(* Logix 5000 Program export KEP; software revision 30.00; part 12 of 15 *)
(* tags used below, declared in another part *)
   B256_CtoE : B256_CtoE;
   B256_CtoS : B256_CtoS;
   B256_EtoC : B256_EtoC;
   B256_StoC_LE : B256_StoC_LE;
   B256_StoSLE : B256_StoSLE;
   EdDSA_INTERNAL : EdDSA_INTERNAL[5];
   EdDSA_STATES : EdDSA_STATECTRL[15];
   InternalFlags : InternalFlags[5];
   InternalFlag_KeyServerIdentityNo : BOOL;
   InternalFlag_KeyServerIdentityYes : BOOL;
   InternalFlag_KsExists : BOOL;
   InternalFlag_KsIDMatchesServer : BOOL;
   InternalFlag_KsPrimeExists : BOOL;
   InternalFlag_KsPrimeIDMatchesServer : BOOL;
   InternalFlag_PowerOnCycle : BOOL;
   MyNodeNumber : DINT;
   POINT_ENC : POINT_ENC;
   POINT_MUL : POINT_MUL;
   PRN : STRING;
   PRNG : PRNG;
   PRNG_Constant : STRING;
   PRNG_Counter : LINT;
   PRNG_Seed : LINT[13];
   ServerNode : INT;
   ServerPriority : DINT[5];
   SignedMsgDest : INT;   // 0=None 1=Server 2=Client 3=All
   Temp_Processor_C1 : DINT[22];
   Temp_Processor_C10 : DINT[22];
   Temp_Processor_C2 : DINT[22];
   Temp_Processor_C3 : DINT[22];
   Temp_Processor_C4 : DINT[22];
   Temp_Processor_C5 : DINT[22];
   Temp_Processor_C6 : DINT[22];
   Temp_Processor_C7 : DINT[22];
   Temp_Processor_C8 : DINT[22];
   Temp_Processor_C9 : DINT[22];
   Temp_Processor_D1 : DINT[43];
   Temp_Processor_E1 : DINT[32];
   Temp_Processor_E2 : DINT[32];
   Temp_Processor_HASH : LINT[8];
   Temp_Processor_L : LINT[4];
   Temp_Processor_MSG : LINT[1600];
   Temp_Processor_P1 : POINT;
   Temp_Processor_P2 : POINT;
   Temp_Processor_P3 : POINT;
   Temp_Processor_P4 : POINT;
   Temp_Processor_S : STRING;
   T_INT1 : INT;
   WorkingNode : DINT;
   NODE : VMAC_DATA_INTERNAL[5];
(* KEP, continued *)

ROUTINE PROCESSOR_STATE1   (* ladder *)
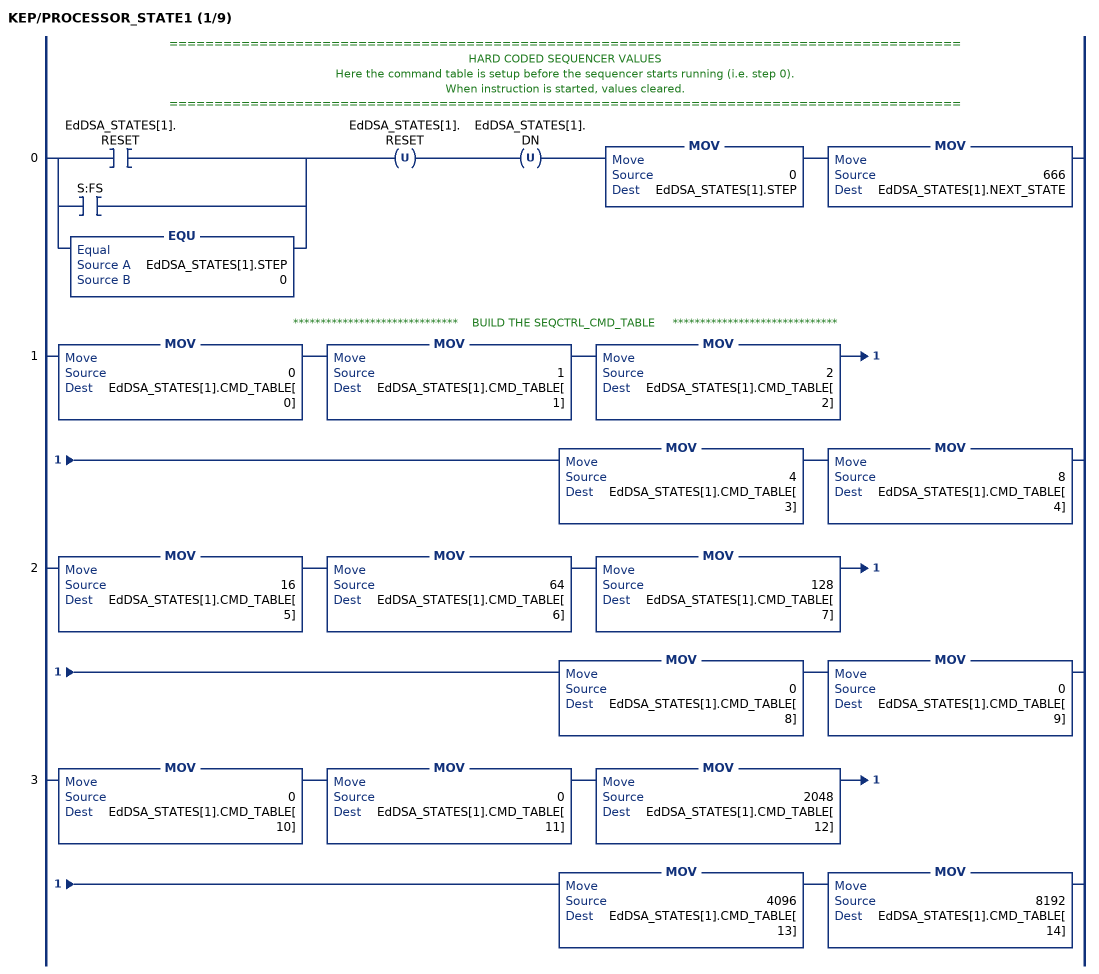
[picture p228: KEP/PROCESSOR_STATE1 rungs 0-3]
   // ========================================================================================
   // HARD CODED SEQUENCER VALUES
   // Here the command table is setup before the sequencer starts running (i.e. step 0).
   // When instruction is started, values cleared.
   // ========================================================================================
   0: [[XIC(EdDSA_STATES[1].RESET) ,XIC(S:FS) ] ,EQU(EdDSA_STATES[1].STEP,0) ]OTU(EdDSA_STATES[1].RESET)OTU(EdDSA_STATES[1].DN)MOV(0,EdDSA_STATES[1].STEP)MOV(666,EdDSA_STATES[1].NEXT_STATE);
   // ******************************    BUILD THE SEQCTRL_CMD_TABLE     ******************************
   1: MOV(0,EdDSA_STATES[1].CMD_TABLE[0])MOV(1,EdDSA_STATES[1].CMD_TABLE[1])MOV(2,EdDSA_STATES[1].CMD_TABLE[2])MOV(4,EdDSA_STATES[1].CMD_TABLE[3])MOV(8,EdDSA_STATES[1].CMD_TABLE[4]);
   2: MOV(16,EdDSA_STATES[1].CMD_TABLE[5])MOV(64,EdDSA_STATES[1].CMD_TABLE[6])MOV(128,EdDSA_STATES[1].CMD_TABLE[7])MOV(0,EdDSA_STATES[1].CMD_TABLE[8])MOV(0,EdDSA_STATES[1].CMD_TABLE[9]);
   3: MOV(0,EdDSA_STATES[1].CMD_TABLE[10])MOV(0,EdDSA_STATES[1].CMD_TABLE[11])MOV(2048,EdDSA_STATES[1].CMD_TABLE[12])MOV(4096,EdDSA_STATES[1].CMD_TABLE[13])MOV(8192,EdDSA_STATES[1].CMD_TABLE[14]);
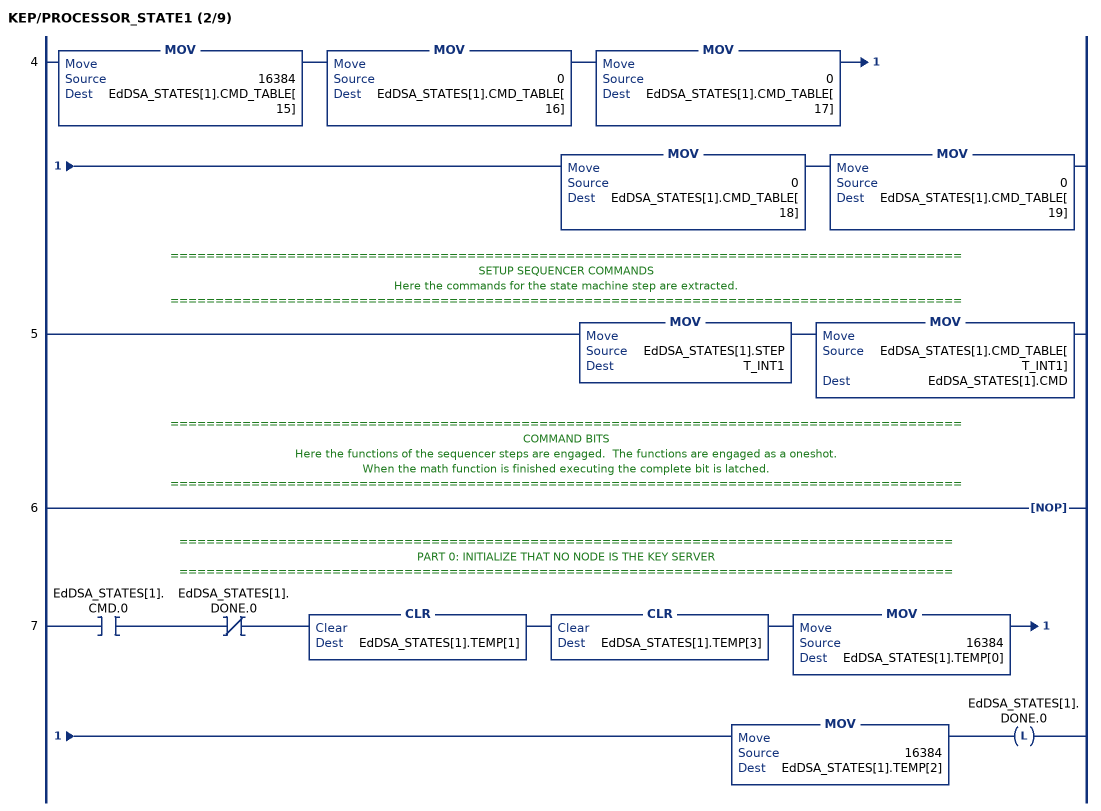
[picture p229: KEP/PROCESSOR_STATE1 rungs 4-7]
   4: MOV(16384,EdDSA_STATES[1].CMD_TABLE[15])MOV(0,EdDSA_STATES[1].CMD_TABLE[16])MOV(0,EdDSA_STATES[1].CMD_TABLE[17])MOV(0,EdDSA_STATES[1].CMD_TABLE[18])MOV(0,EdDSA_STATES[1].CMD_TABLE[19]);
   // ========================================================================================
   // SETUP SEQUENCER COMMANDS
   // Here the commands for the state machine step are extracted.
   // ========================================================================================
   5: MOV(EdDSA_STATES[1].STEP,T_INT1)MOV(EdDSA_STATES[1].CMD_TABLE[T_INT1],EdDSA_STATES[1].CMD);
   // ========================================================================================
   // COMMAND BITS
   // Here the functions of the sequencer steps are engaged.  The functions are engaged as a oneshot.
   // When the math function is finished executing the complete bit is latched.
   // ========================================================================================
   6: NOP();
   // ======================================================================================
   // PART 0: INITIALIZE THAT NO NODE IS THE KEY SERVER
   // ======================================================================================
   7: XIC(EdDSA_STATES[1].CMD.0)XIO(EdDSA_STATES[1].DONE.0)CLR(EdDSA_STATES[1].TEMP[1])CLR(EdDSA_STATES[1].TEMP[3])MOV(16384,EdDSA_STATES[1].TEMP[0])MOV(16384,EdDSA_STATES[1].TEMP[2])OTL(EdDSA_STATES[1].DONE.0);
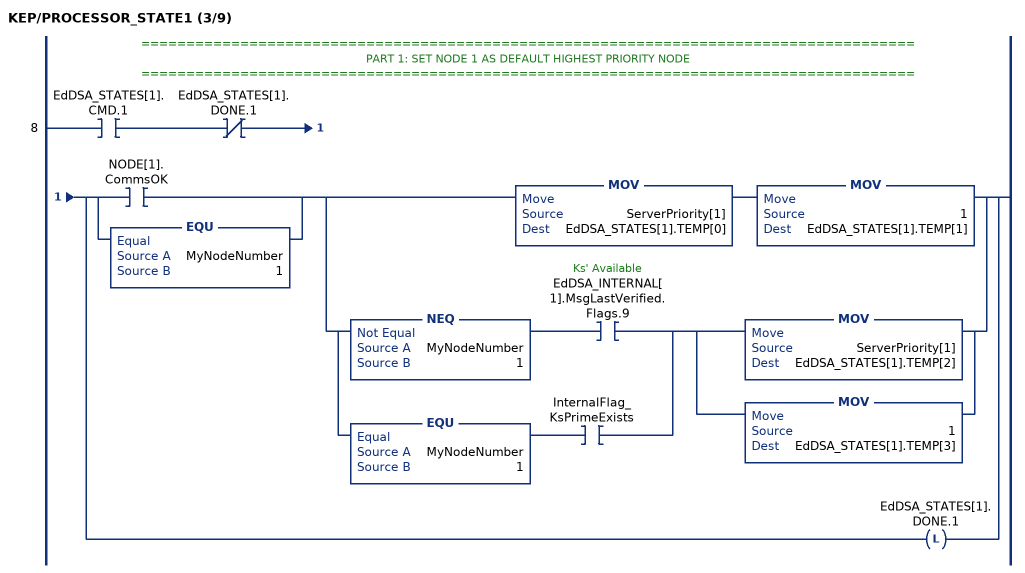
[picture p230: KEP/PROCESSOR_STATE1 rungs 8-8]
   // ======================================================================================
   // PART 1: SET NODE 1 AS DEFAULT HIGHEST PRIORITY NODE
   // ======================================================================================
   8: XIC(EdDSA_STATES[1].CMD.1)XIO(EdDSA_STATES[1].DONE.1)[[XIC(NODE[1].CommsOK) ,EQU(MyNodeNumber,1) ] [MOV(ServerPriority[1],EdDSA_STATES[1].TEMP[0]) MOV(1,EdDSA_STATES[1].TEMP[1]) ,[NEQ(MyNodeNumber,1) XIC(EdDSA_INTERNAL[1].MsgLastVerified.Flags.9) ,EQU(MyNodeNumber,1) XIC(InternalFlag_KsPrimeExists) ] [MOV(ServerPriority[1],EdDSA_STATES[1].TEMP[2]) ,MOV(1,EdDSA_STATES[1].TEMP[3]) ] ] ,OTL(EdDSA_STATES[1].DONE.1) ];
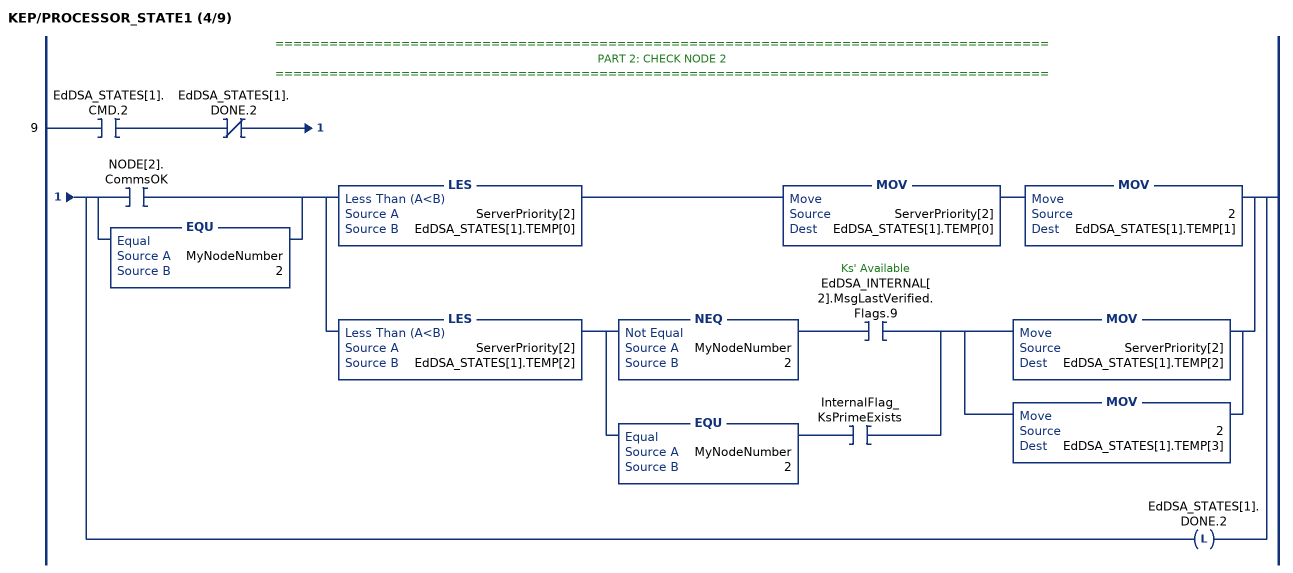
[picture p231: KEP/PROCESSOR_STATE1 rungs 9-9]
   // ======================================================================================
   // PART 2: CHECK NODE 2
   // ======================================================================================
   9: XIC(EdDSA_STATES[1].CMD.2)XIO(EdDSA_STATES[1].DONE.2)[[XIC(NODE[2].CommsOK) ,EQU(MyNodeNumber,2) ] [LES(ServerPriority[2],EdDSA_STATES[1].TEMP[0]) MOV(ServerPriority[2],EdDSA_STATES[1].TEMP[0]) MOV(2,EdDSA_STATES[1].TEMP[1]) ,LES(ServerPriority[2],EdDSA_STATES[1].TEMP[2]) [NEQ(MyNodeNumber,2) XIC(EdDSA_INTERNAL[2].MsgLastVerified.Flags.9) ,EQU(MyNodeNumber,2) XIC(InternalFlag_KsPrimeExists) ] [MOV(ServerPriority[2],EdDSA_STATES[1].TEMP[2]) ,MOV(2,EdDSA_STATES[1].TEMP[3]) ] ] ,OTL(EdDSA_STATES[1].DONE.2) ];
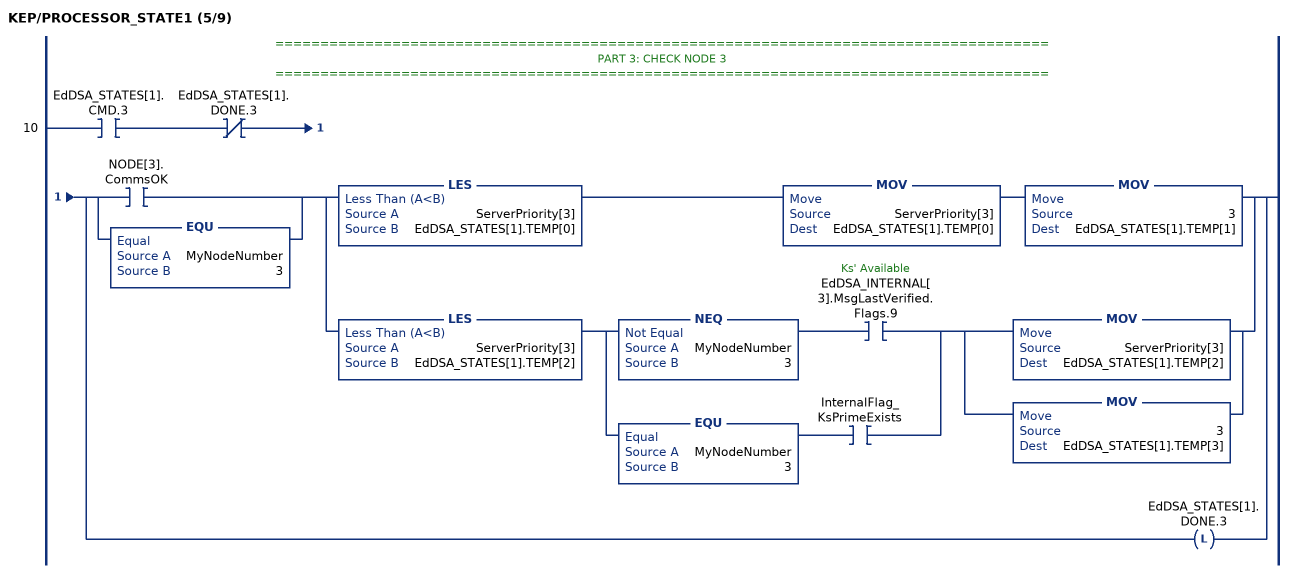
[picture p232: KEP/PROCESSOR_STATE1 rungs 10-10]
   // ======================================================================================
   // PART 3: CHECK NODE 3
   // ======================================================================================
   10: XIC(EdDSA_STATES[1].CMD.3)XIO(EdDSA_STATES[1].DONE.3)[[XIC(NODE[3].CommsOK) ,EQU(MyNodeNumber,3) ] [LES(ServerPriority[3],EdDSA_STATES[1].TEMP[0]) MOV(ServerPriority[3],EdDSA_STATES[1].TEMP[0]) MOV(3,EdDSA_STATES[1].TEMP[1]) ,LES(ServerPriority[3],EdDSA_STATES[1].TEMP[2]) [NEQ(MyNodeNumber,3) XIC(EdDSA_INTERNAL[3].MsgLastVerified.Flags.9) ,EQU(MyNodeNumber,3) XIC(InternalFlag_KsPrimeExists) ] [MOV(ServerPriority[3],EdDSA_STATES[1].TEMP[2]) ,MOV(3,EdDSA_STATES[1].TEMP[3]) ] ] ,OTL(EdDSA_STATES[1].DONE.3) ];
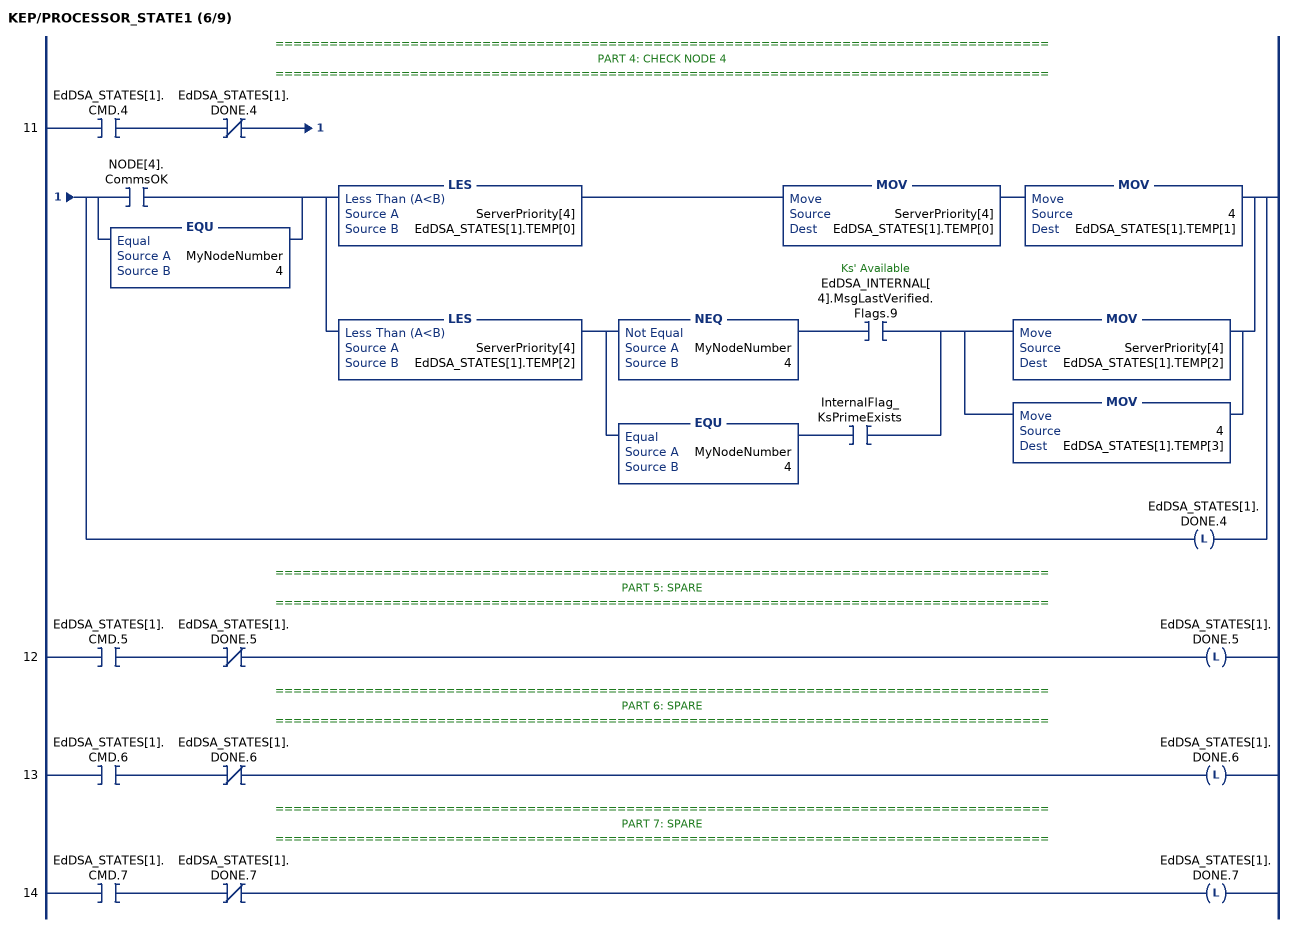
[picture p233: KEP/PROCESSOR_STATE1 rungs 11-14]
   // ======================================================================================
   // PART 4: CHECK NODE 4
   // ======================================================================================
   11: XIC(EdDSA_STATES[1].CMD.4)XIO(EdDSA_STATES[1].DONE.4)[[XIC(NODE[4].CommsOK) ,EQU(MyNodeNumber,4) ] [LES(ServerPriority[4],EdDSA_STATES[1].TEMP[0]) MOV(ServerPriority[4],EdDSA_STATES[1].TEMP[0]) MOV(4,EdDSA_STATES[1].TEMP[1]) ,LES(ServerPriority[4],EdDSA_STATES[1].TEMP[2]) [NEQ(MyNodeNumber,4) XIC(EdDSA_INTERNAL[4].MsgLastVerified.Flags.9) ,EQU(MyNodeNumber,4) XIC(InternalFlag_KsPrimeExists) ] [MOV(ServerPriority[4],EdDSA_STATES[1].TEMP[2]) ,MOV(4,EdDSA_STATES[1].TEMP[3]) ] ] ,OTL(EdDSA_STATES[1].DONE.4) ];
   // ======================================================================================
   // PART 5: SPARE
   // ======================================================================================
   12: XIC(EdDSA_STATES[1].CMD.5)XIO(EdDSA_STATES[1].DONE.5)OTL(EdDSA_STATES[1].DONE.5);
   // ======================================================================================
   // PART 6: SPARE
   // ======================================================================================
   13: XIC(EdDSA_STATES[1].CMD.6)XIO(EdDSA_STATES[1].DONE.6)OTL(EdDSA_STATES[1].DONE.6);
   // ======================================================================================
   // PART 7: SPARE
   // ======================================================================================
   14: XIC(EdDSA_STATES[1].CMD.7)XIO(EdDSA_STATES[1].DONE.7)OTL(EdDSA_STATES[1].DONE.7);
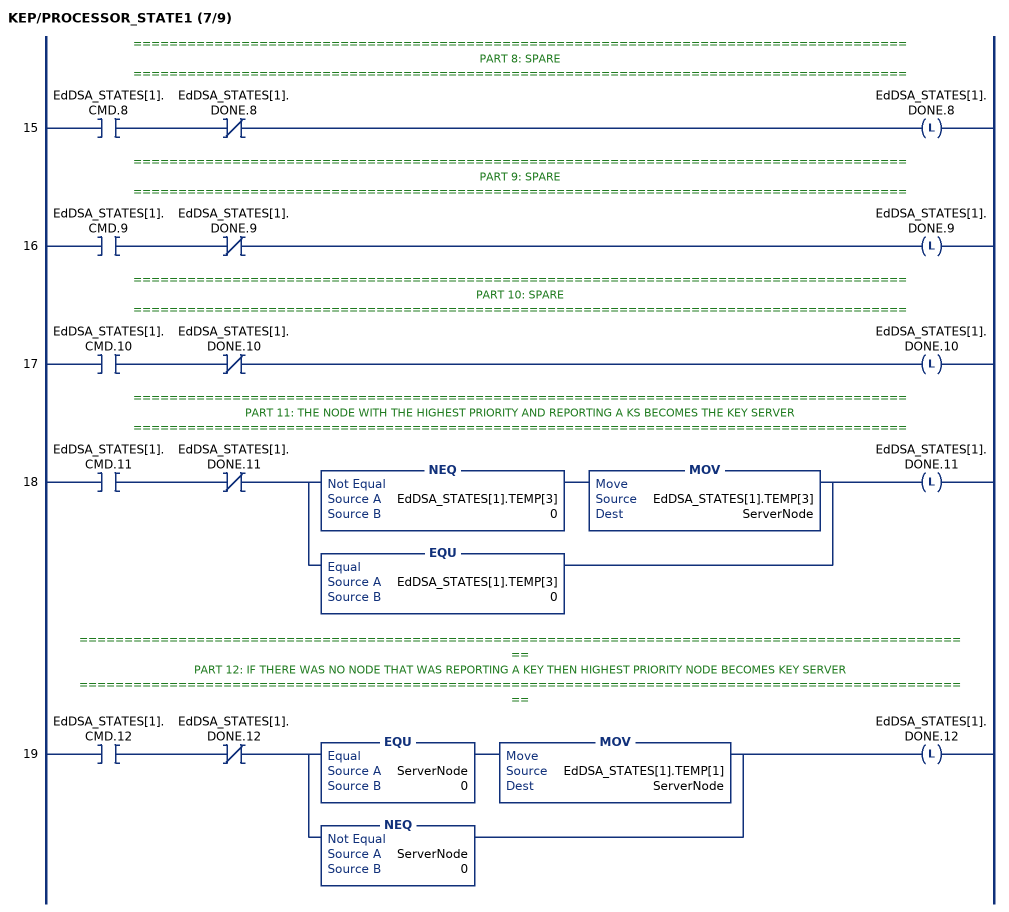
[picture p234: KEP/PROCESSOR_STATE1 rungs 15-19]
   // ======================================================================================
   // PART 8: SPARE
   // ======================================================================================
   15: XIC(EdDSA_STATES[1].CMD.8)XIO(EdDSA_STATES[1].DONE.8)OTL(EdDSA_STATES[1].DONE.8);
   // ======================================================================================
   // PART 9: SPARE
   // ======================================================================================
   16: XIC(EdDSA_STATES[1].CMD.9)XIO(EdDSA_STATES[1].DONE.9)OTL(EdDSA_STATES[1].DONE.9);
   // ======================================================================================
   // PART 10: SPARE
   // ======================================================================================
   17: XIC(EdDSA_STATES[1].CMD.10)XIO(EdDSA_STATES[1].DONE.10)OTL(EdDSA_STATES[1].DONE.10);
   // ======================================================================================
   // PART 11: THE NODE WITH THE HIGHEST PRIORITY AND REPORTING A KS BECOMES THE KEY SERVER
   // ======================================================================================
   18: XIC(EdDSA_STATES[1].CMD.11)XIO(EdDSA_STATES[1].DONE.11)[NEQ(EdDSA_STATES[1].TEMP[3],0) MOV(EdDSA_STATES[1].TEMP[3],ServerNode) ,EQU(EdDSA_STATES[1].TEMP[3],0) ]OTL(EdDSA_STATES[1].DONE.11);
   // ====================================================================================================
   // PART 12: IF THERE WAS NO NODE THAT WAS REPORTING A KEY THEN HIGHEST PRIORITY NODE BECOMES KEY SERVER
   // ====================================================================================================
   19: XIC(EdDSA_STATES[1].CMD.12)XIO(EdDSA_STATES[1].DONE.12)[EQU(ServerNode,0) MOV(EdDSA_STATES[1].TEMP[1],ServerNode) ,NEQ(ServerNode,0) ]OTL(EdDSA_STATES[1].DONE.12);
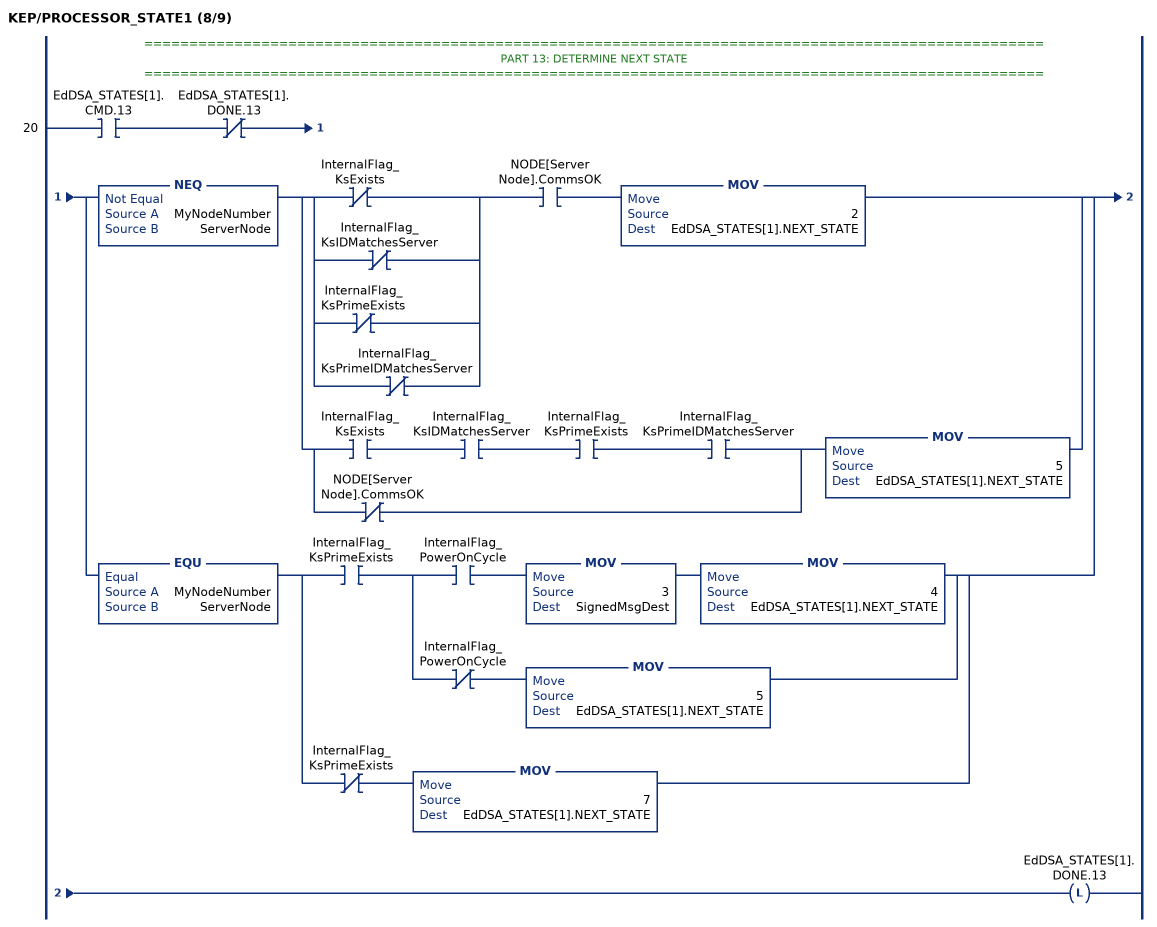
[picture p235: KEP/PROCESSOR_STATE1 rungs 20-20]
   // ====================================================================================================
   // PART 13: DETERMINE NEXT STATE
   // ====================================================================================================
   20: XIC(EdDSA_STATES[1].CMD.13)XIO(EdDSA_STATES[1].DONE.13)[NEQ(MyNodeNumber,ServerNode) [[XIO(InternalFlag_KsExists) ,XIO(InternalFlag_KsIDMatchesServer) ,XIO(InternalFlag_KsPrimeExists) ,XIO(InternalFlag_KsPrimeIDMatchesServer) ] XIC(NODE[ServerNode].CommsOK) MOV(2,EdDSA_STATES[1].NEXT_STATE) ,[XIC(InternalFlag_KsExists) XIC(InternalFlag_KsIDMatchesServer) XIC(InternalFlag_KsPrimeExists) XIC(InternalFlag_KsPrimeIDMatchesServer) ,XIO(NODE[ServerNode].CommsOK) ] MOV(5,EdDSA_STATES[1].NEXT_STATE) ] ,EQU(MyNodeNumber,ServerNode) [XIC(InternalFlag_KsPrimeExists) [XIC(InternalFlag_PowerOnCycle) MOV(3,SignedMsgDest) MOV(4,EdDSA_STATES[1].NEXT_STATE) ,XIO(InternalFlag_PowerOnCycle) MOV(5,EdDSA_STATES[1].NEXT_STATE) ] ,XIO(InternalFlag_KsPrimeExists) MOV(7,EdDSA_STATES[1].NEXT_STATE) ] ]OTL(EdDSA_STATES[1].DONE.13);
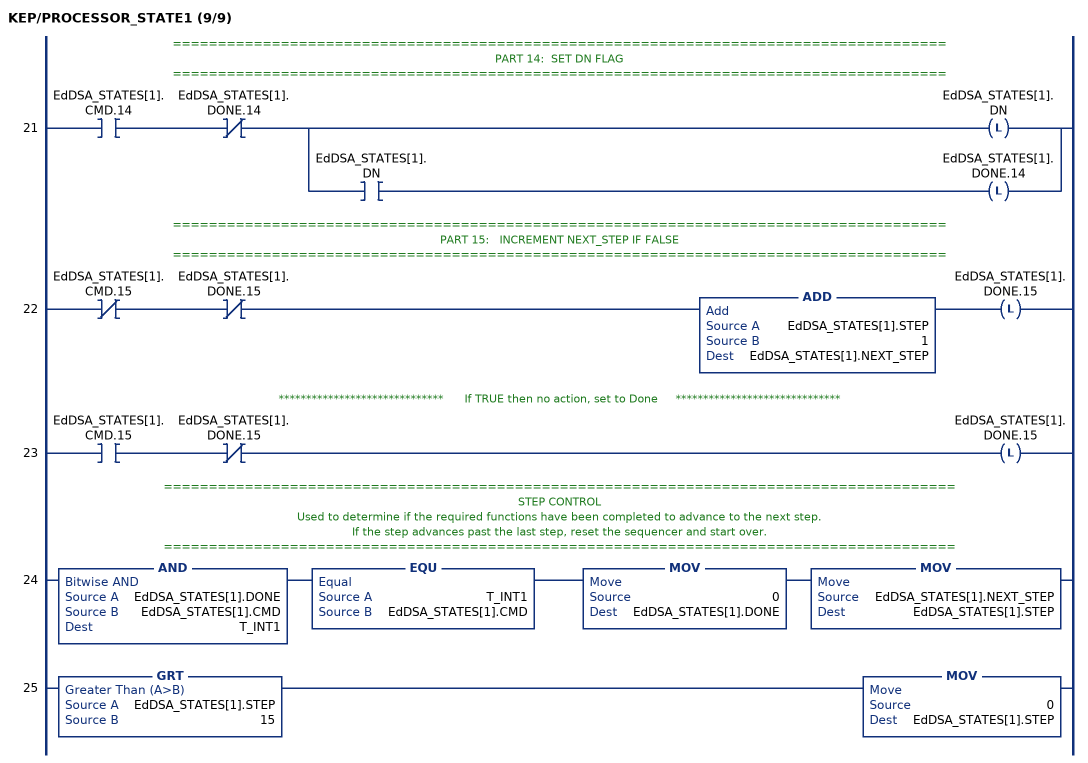
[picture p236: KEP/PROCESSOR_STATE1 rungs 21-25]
   // ======================================================================================
   // PART 14:  SET DN FLAG
   // ======================================================================================
   21: XIC(EdDSA_STATES[1].CMD.14)XIO(EdDSA_STATES[1].DONE.14)[OTL(EdDSA_STATES[1].DN) ,XIC(EdDSA_STATES[1].DN) OTL(EdDSA_STATES[1].DONE.14) ];
   // ======================================================================================
   // PART 15:   INCREMENT NEXT_STEP IF FALSE
   // ======================================================================================
   22: XIO(EdDSA_STATES[1].CMD.15)XIO(EdDSA_STATES[1].DONE.15)ADD(EdDSA_STATES[1].STEP,1,EdDSA_STATES[1].NEXT_STEP)OTL(EdDSA_STATES[1].DONE.15);
   // ******************************      If TRUE then no action, set to Done     ******************************
   23: XIC(EdDSA_STATES[1].CMD.15)XIO(EdDSA_STATES[1].DONE.15)OTL(EdDSA_STATES[1].DONE.15);
   // ========================================================================================
   // STEP CONTROL
   // Used to determine if the required functions have been completed to advance to the next step.
   // If the step advances past the last step, reset the sequencer and start over.
   // ========================================================================================
   24: AND(EdDSA_STATES[1].DONE,EdDSA_STATES[1].CMD,T_INT1)EQU(T_INT1,EdDSA_STATES[1].CMD)MOV(0,EdDSA_STATES[1].DONE)MOV(EdDSA_STATES[1].NEXT_STEP,EdDSA_STATES[1].STEP);
   25: GRT(EdDSA_STATES[1].STEP,15)MOV(0,EdDSA_STATES[1].STEP);
END_ROUTINE

ROUTINE PROCESSOR_STATE2   (* ladder *)
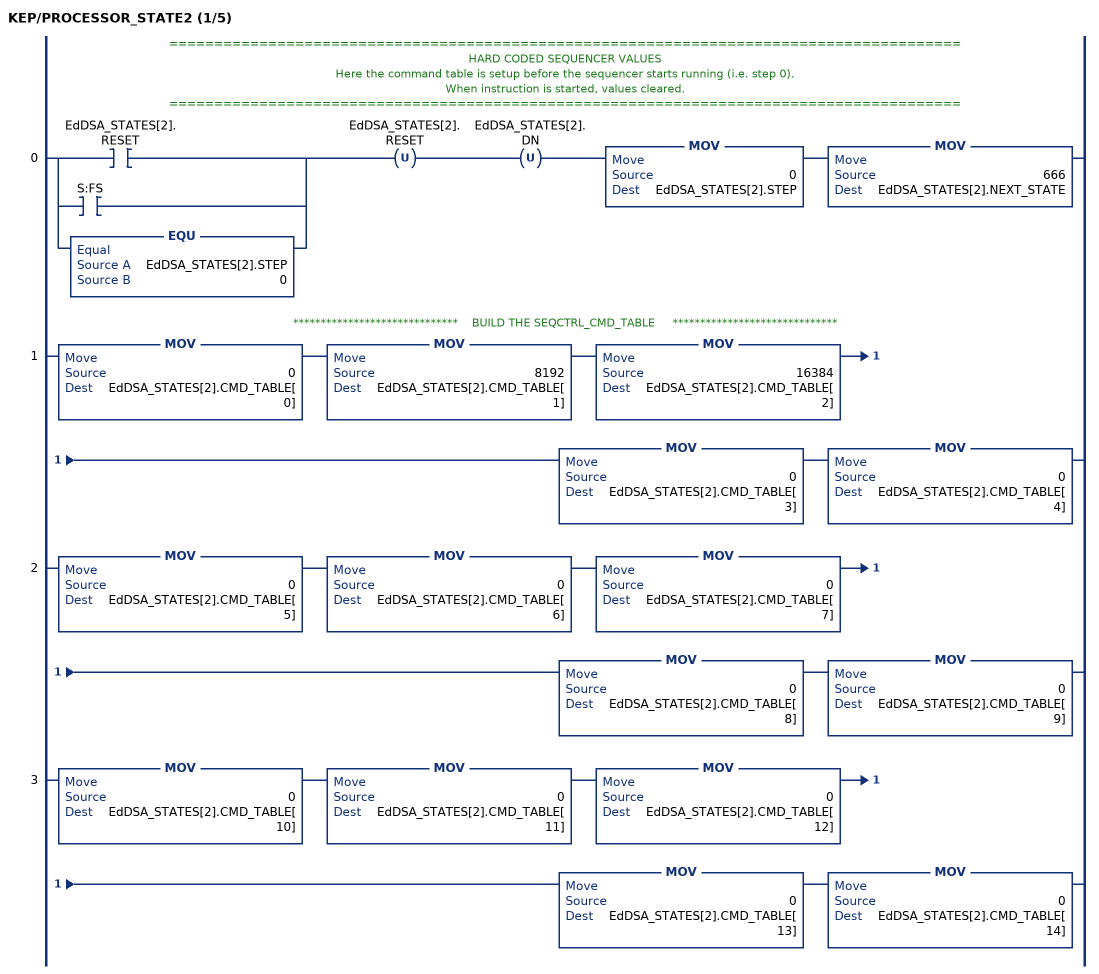
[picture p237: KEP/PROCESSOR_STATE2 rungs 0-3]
   // ========================================================================================
   // HARD CODED SEQUENCER VALUES
   // Here the command table is setup before the sequencer starts running (i.e. step 0).
   // When instruction is started, values cleared.
   // ========================================================================================
   0: [[XIC(EdDSA_STATES[2].RESET) ,XIC(S:FS) ] ,EQU(EdDSA_STATES[2].STEP,0) ]OTU(EdDSA_STATES[2].RESET)OTU(EdDSA_STATES[2].DN)MOV(0,EdDSA_STATES[2].STEP)MOV(666,EdDSA_STATES[2].NEXT_STATE);
   // ******************************    BUILD THE SEQCTRL_CMD_TABLE     ******************************
   1: MOV(0,EdDSA_STATES[2].CMD_TABLE[0])MOV(8192,EdDSA_STATES[2].CMD_TABLE[1])MOV(16384,EdDSA_STATES[2].CMD_TABLE[2])MOV(0,EdDSA_STATES[2].CMD_TABLE[3])MOV(0,EdDSA_STATES[2].CMD_TABLE[4]);
   2: MOV(0,EdDSA_STATES[2].CMD_TABLE[5])MOV(0,EdDSA_STATES[2].CMD_TABLE[6])MOV(0,EdDSA_STATES[2].CMD_TABLE[7])MOV(0,EdDSA_STATES[2].CMD_TABLE[8])MOV(0,EdDSA_STATES[2].CMD_TABLE[9]);
   3: MOV(0,EdDSA_STATES[2].CMD_TABLE[10])MOV(0,EdDSA_STATES[2].CMD_TABLE[11])MOV(0,EdDSA_STATES[2].CMD_TABLE[12])MOV(0,EdDSA_STATES[2].CMD_TABLE[13])MOV(0,EdDSA_STATES[2].CMD_TABLE[14]);
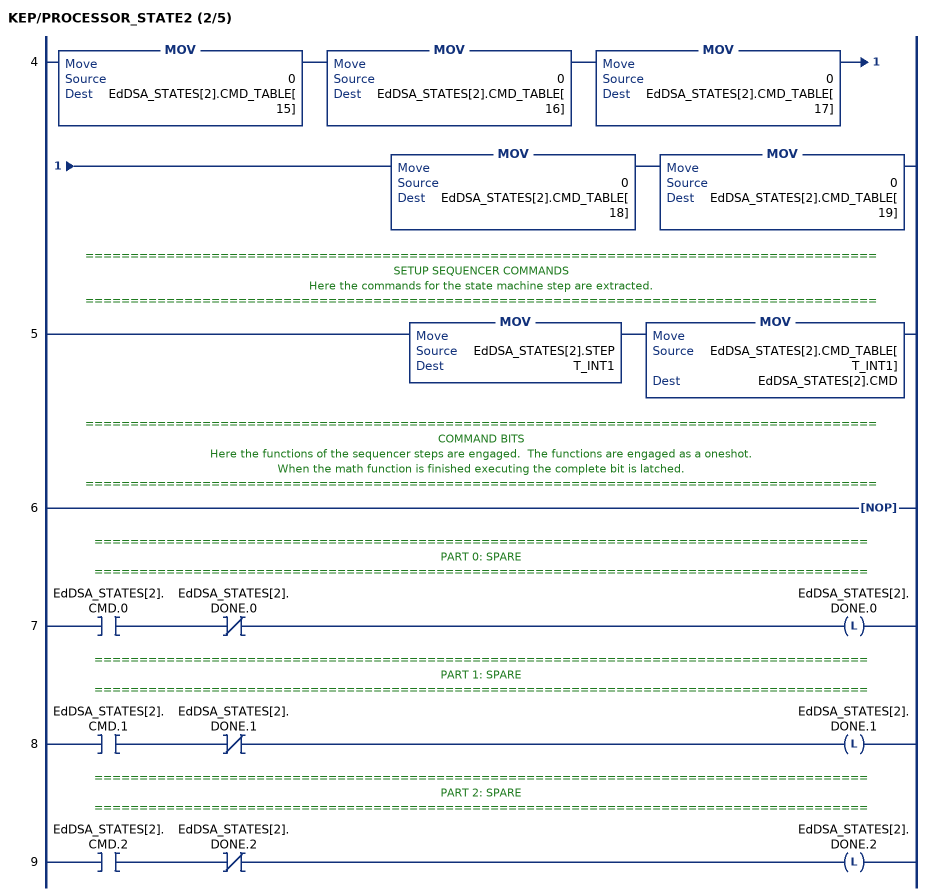
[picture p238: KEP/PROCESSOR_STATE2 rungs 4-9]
   4: MOV(0,EdDSA_STATES[2].CMD_TABLE[15])MOV(0,EdDSA_STATES[2].CMD_TABLE[16])MOV(0,EdDSA_STATES[2].CMD_TABLE[17])MOV(0,EdDSA_STATES[2].CMD_TABLE[18])MOV(0,EdDSA_STATES[2].CMD_TABLE[19]);
   // ========================================================================================
   // SETUP SEQUENCER COMMANDS
   // Here the commands for the state machine step are extracted.
   // ========================================================================================
   5: MOV(EdDSA_STATES[2].STEP,T_INT1)MOV(EdDSA_STATES[2].CMD_TABLE[T_INT1],EdDSA_STATES[2].CMD);
   // ========================================================================================
   // COMMAND BITS
   // Here the functions of the sequencer steps are engaged.  The functions are engaged as a oneshot.
   // When the math function is finished executing the complete bit is latched.
   // ========================================================================================
   6: NOP();
   // ======================================================================================
   // PART 0: SPARE
   // ======================================================================================
   7: XIC(EdDSA_STATES[2].CMD.0)XIO(EdDSA_STATES[2].DONE.0)OTL(EdDSA_STATES[2].DONE.0);
   // ======================================================================================
   // PART 1: SPARE
   // ======================================================================================
   8: XIC(EdDSA_STATES[2].CMD.1)XIO(EdDSA_STATES[2].DONE.1)OTL(EdDSA_STATES[2].DONE.1);
   // ======================================================================================
   // PART 2: SPARE
   // ======================================================================================
   9: XIC(EdDSA_STATES[2].CMD.2)XIO(EdDSA_STATES[2].DONE.2)OTL(EdDSA_STATES[2].DONE.2);
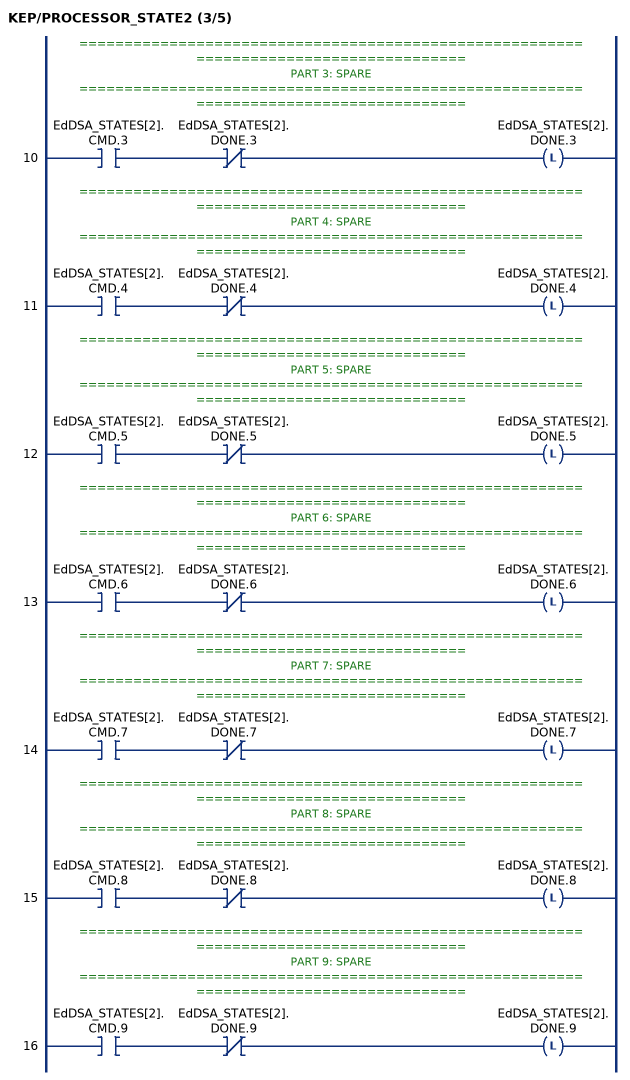
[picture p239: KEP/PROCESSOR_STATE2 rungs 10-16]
   // ======================================================================================
   // PART 3: SPARE
   // ======================================================================================
   10: XIC(EdDSA_STATES[2].CMD.3)XIO(EdDSA_STATES[2].DONE.3)OTL(EdDSA_STATES[2].DONE.3);
   // ======================================================================================
   // PART 4: SPARE
   // ======================================================================================
   11: XIC(EdDSA_STATES[2].CMD.4)XIO(EdDSA_STATES[2].DONE.4)OTL(EdDSA_STATES[2].DONE.4);
   // ======================================================================================
   // PART 5: SPARE
   // ======================================================================================
   12: XIC(EdDSA_STATES[2].CMD.5)XIO(EdDSA_STATES[2].DONE.5)OTL(EdDSA_STATES[2].DONE.5);
   // ======================================================================================
   // PART 6: SPARE
   // ======================================================================================
   13: XIC(EdDSA_STATES[2].CMD.6)XIO(EdDSA_STATES[2].DONE.6)OTL(EdDSA_STATES[2].DONE.6);
   // ======================================================================================
   // PART 7: SPARE
   // ======================================================================================
   14: XIC(EdDSA_STATES[2].CMD.7)XIO(EdDSA_STATES[2].DONE.7)OTL(EdDSA_STATES[2].DONE.7);
   // ======================================================================================
   // PART 8: SPARE
   // ======================================================================================
   15: XIC(EdDSA_STATES[2].CMD.8)XIO(EdDSA_STATES[2].DONE.8)OTL(EdDSA_STATES[2].DONE.8);
   // ======================================================================================
   // PART 9: SPARE
   // ======================================================================================
   16: XIC(EdDSA_STATES[2].CMD.9)XIO(EdDSA_STATES[2].DONE.9)OTL(EdDSA_STATES[2].DONE.9);
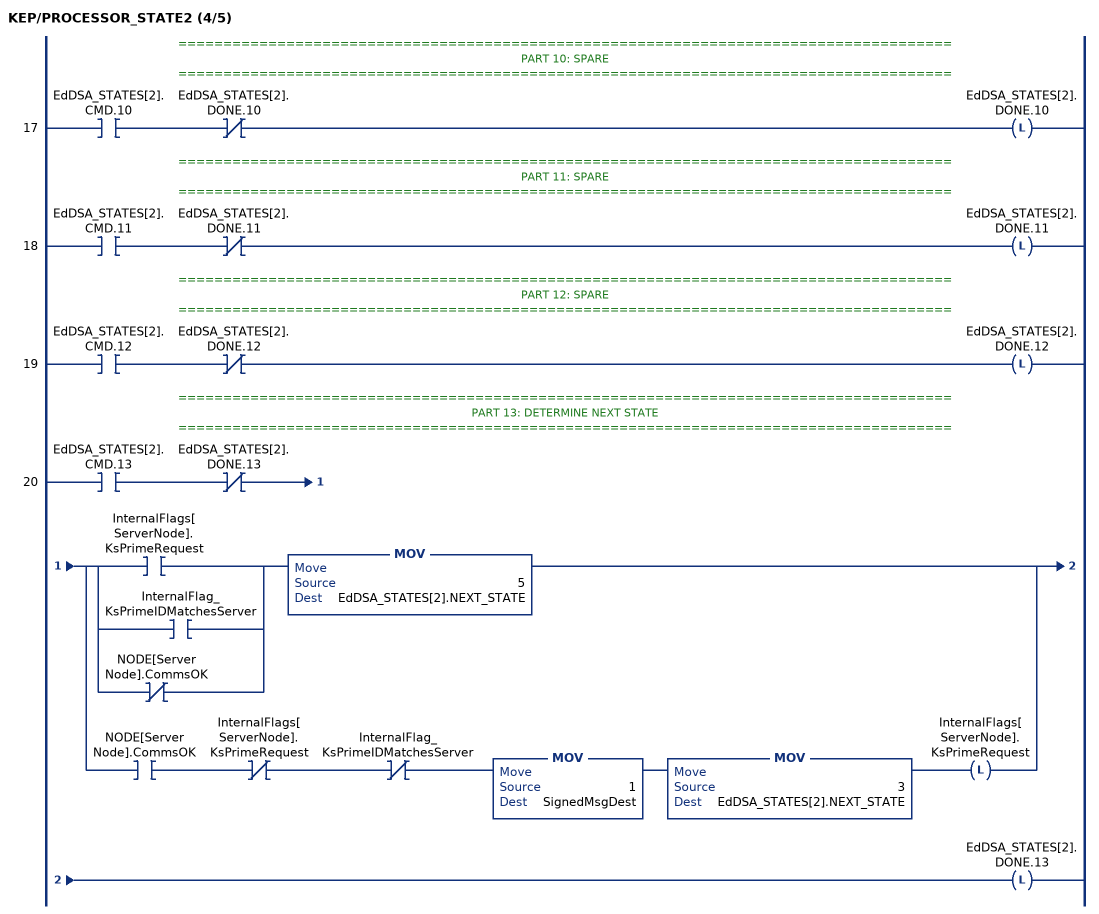
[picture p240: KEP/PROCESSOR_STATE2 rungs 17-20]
   // ======================================================================================
   // PART 10: SPARE
   // ======================================================================================
   17: XIC(EdDSA_STATES[2].CMD.10)XIO(EdDSA_STATES[2].DONE.10)OTL(EdDSA_STATES[2].DONE.10);
   // ======================================================================================
   // PART 11: SPARE
   // ======================================================================================
   18: XIC(EdDSA_STATES[2].CMD.11)XIO(EdDSA_STATES[2].DONE.11)OTL(EdDSA_STATES[2].DONE.11);
   // ======================================================================================
   // PART 12: SPARE
   // ======================================================================================
   19: XIC(EdDSA_STATES[2].CMD.12)XIO(EdDSA_STATES[2].DONE.12)OTL(EdDSA_STATES[2].DONE.12);
   // ======================================================================================
   // PART 13: DETERMINE NEXT STATE
   // ======================================================================================
   20: XIC(EdDSA_STATES[2].CMD.13)XIO(EdDSA_STATES[2].DONE.13)[[XIC(InternalFlags[ServerNode].KsPrimeRequest) ,XIC(InternalFlag_KsPrimeIDMatchesServer) ,XIO(NODE[ServerNode].CommsOK) ] MOV(5,EdDSA_STATES[2].NEXT_STATE) ,XIC(NODE[ServerNode].CommsOK) XIO(InternalFlags[ServerNode].KsPrimeRequest) XIO(InternalFlag_KsPrimeIDMatchesServer) MOV(1,SignedMsgDest) MOV(3,EdDSA_STATES[2].NEXT_STATE) OTL(InternalFlags[ServerNode].KsPrimeRequest) ]OTL(EdDSA_STATES[2].DONE.13);
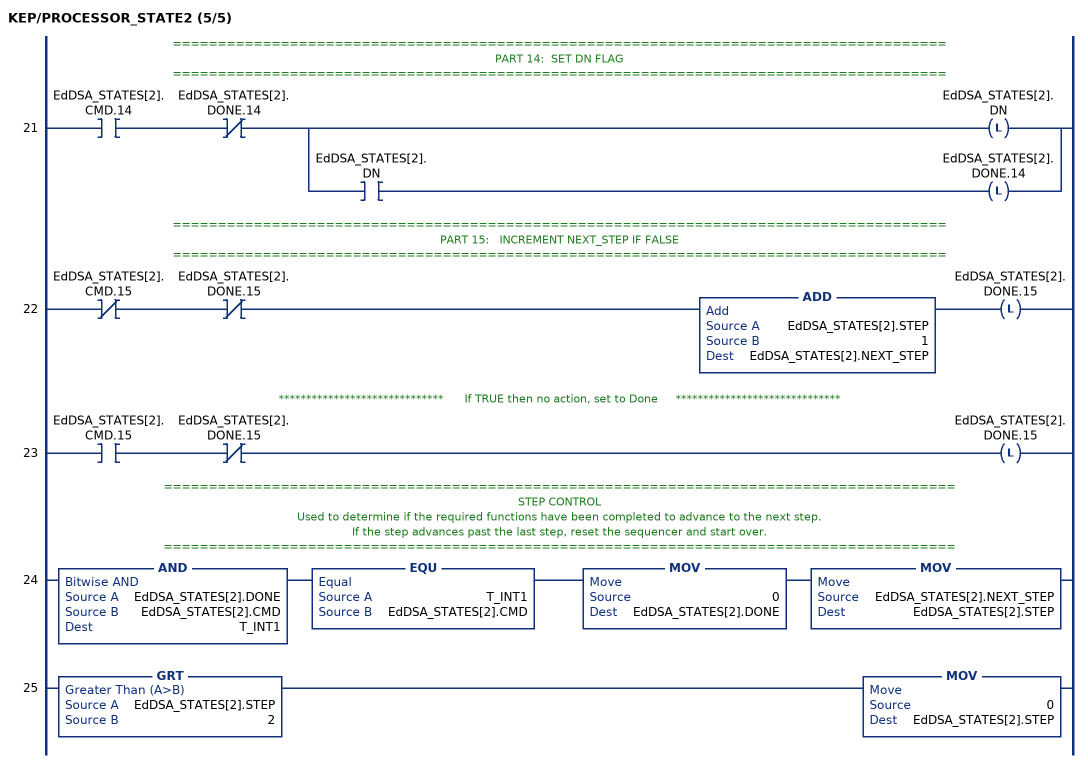
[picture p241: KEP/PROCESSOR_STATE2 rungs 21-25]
   // ======================================================================================
   // PART 14:  SET DN FLAG
   // ======================================================================================
   21: XIC(EdDSA_STATES[2].CMD.14)XIO(EdDSA_STATES[2].DONE.14)[OTL(EdDSA_STATES[2].DN) ,XIC(EdDSA_STATES[2].DN) OTL(EdDSA_STATES[2].DONE.14) ];
   // ======================================================================================
   // PART 15:   INCREMENT NEXT_STEP IF FALSE
   // ======================================================================================
   22: XIO(EdDSA_STATES[2].CMD.15)XIO(EdDSA_STATES[2].DONE.15)ADD(EdDSA_STATES[2].STEP,1,EdDSA_STATES[2].NEXT_STEP)OTL(EdDSA_STATES[2].DONE.15);
   // ******************************      If TRUE then no action, set to Done     ******************************
   23: XIC(EdDSA_STATES[2].CMD.15)XIO(EdDSA_STATES[2].DONE.15)OTL(EdDSA_STATES[2].DONE.15);
   // ========================================================================================
   // STEP CONTROL
   // Used to determine if the required functions have been completed to advance to the next step.
   // If the step advances past the last step, reset the sequencer and start over.
   // ========================================================================================
   24: AND(EdDSA_STATES[2].DONE,EdDSA_STATES[2].CMD,T_INT1)EQU(T_INT1,EdDSA_STATES[2].CMD)MOV(0,EdDSA_STATES[2].DONE)MOV(EdDSA_STATES[2].NEXT_STEP,EdDSA_STATES[2].STEP);
   25: GRT(EdDSA_STATES[2].STEP,2)MOV(0,EdDSA_STATES[2].STEP);
END_ROUTINE

ROUTINE PROCESSOR_STATE3   (* ladder *)
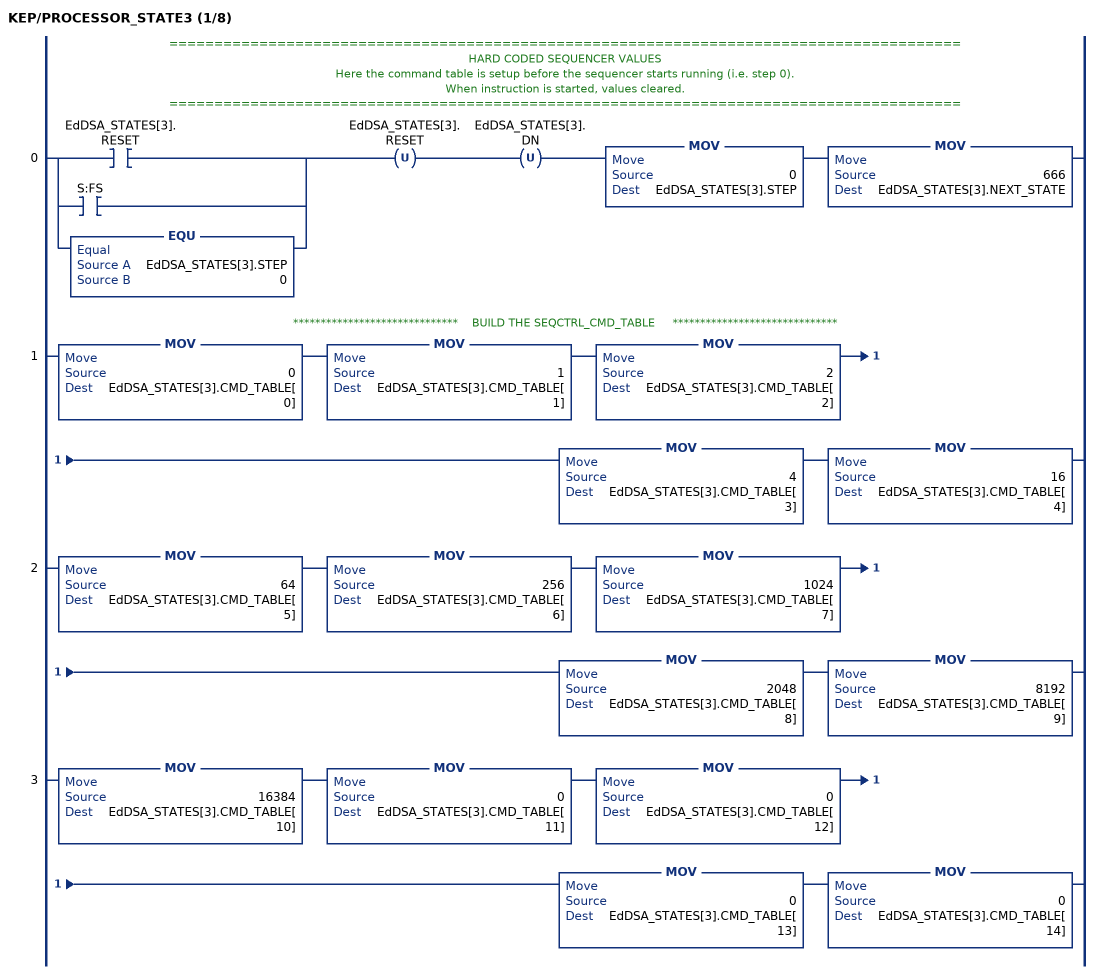
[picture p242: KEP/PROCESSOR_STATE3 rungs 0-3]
   // ========================================================================================
   // HARD CODED SEQUENCER VALUES
   // Here the command table is setup before the sequencer starts running (i.e. step 0).
   // When instruction is started, values cleared.
   // ========================================================================================
   0: [[XIC(EdDSA_STATES[3].RESET) ,XIC(S:FS) ] ,EQU(EdDSA_STATES[3].STEP,0) ]OTU(EdDSA_STATES[3].RESET)OTU(EdDSA_STATES[3].DN)MOV(0,EdDSA_STATES[3].STEP)MOV(666,EdDSA_STATES[3].NEXT_STATE);
   // ******************************    BUILD THE SEQCTRL_CMD_TABLE     ******************************
   1: MOV(0,EdDSA_STATES[3].CMD_TABLE[0])MOV(1,EdDSA_STATES[3].CMD_TABLE[1])MOV(2,EdDSA_STATES[3].CMD_TABLE[2])MOV(4,EdDSA_STATES[3].CMD_TABLE[3])MOV(16,EdDSA_STATES[3].CMD_TABLE[4]);
   2: MOV(64,EdDSA_STATES[3].CMD_TABLE[5])MOV(256,EdDSA_STATES[3].CMD_TABLE[6])MOV(1024,EdDSA_STATES[3].CMD_TABLE[7])MOV(2048,EdDSA_STATES[3].CMD_TABLE[8])MOV(8192,EdDSA_STATES[3].CMD_TABLE[9]);
   3: MOV(16384,EdDSA_STATES[3].CMD_TABLE[10])MOV(0,EdDSA_STATES[3].CMD_TABLE[11])MOV(0,EdDSA_STATES[3].CMD_TABLE[12])MOV(0,EdDSA_STATES[3].CMD_TABLE[13])MOV(0,EdDSA_STATES[3].CMD_TABLE[14]);
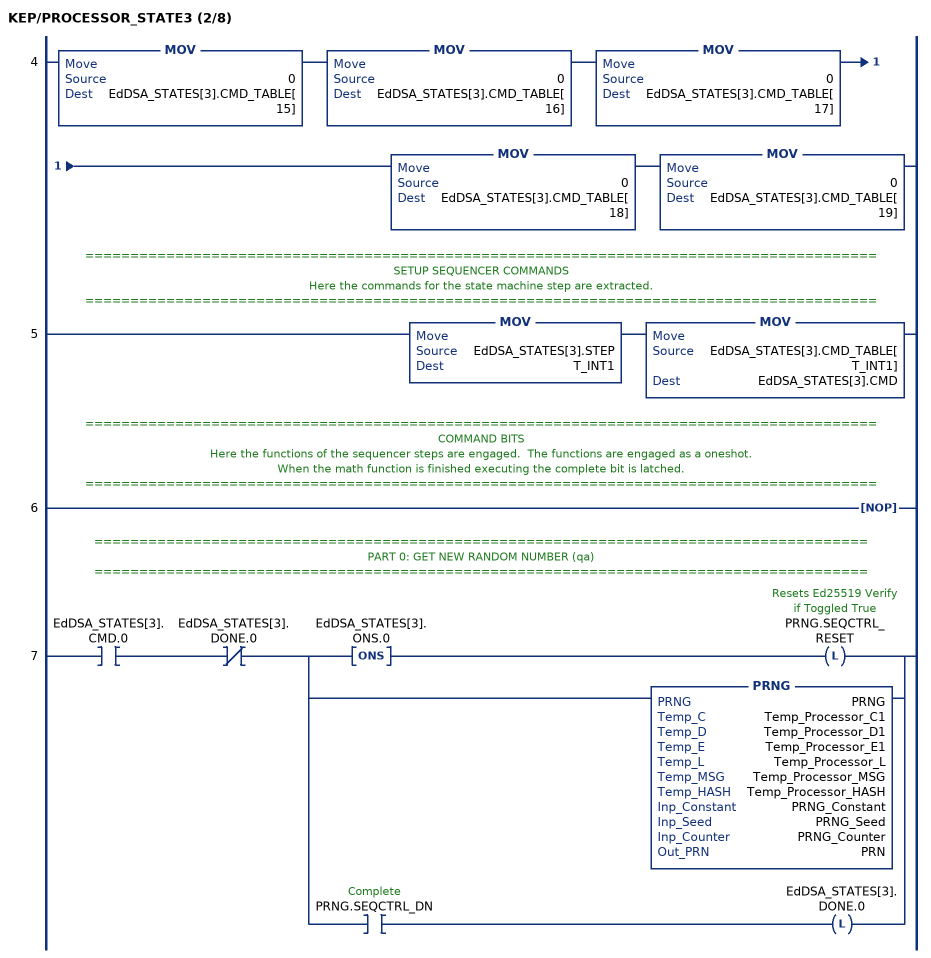
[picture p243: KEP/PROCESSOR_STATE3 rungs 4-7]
   4: MOV(0,EdDSA_STATES[3].CMD_TABLE[15])MOV(0,EdDSA_STATES[3].CMD_TABLE[16])MOV(0,EdDSA_STATES[3].CMD_TABLE[17])MOV(0,EdDSA_STATES[3].CMD_TABLE[18])MOV(0,EdDSA_STATES[3].CMD_TABLE[19]);
   // ========================================================================================
   // SETUP SEQUENCER COMMANDS
   // Here the commands for the state machine step are extracted.
   // ========================================================================================
   5: MOV(EdDSA_STATES[3].STEP,T_INT1)MOV(EdDSA_STATES[3].CMD_TABLE[T_INT1],EdDSA_STATES[3].CMD);
   // ========================================================================================
   // COMMAND BITS
   // Here the functions of the sequencer steps are engaged.  The functions are engaged as a oneshot.
   // When the math function is finished executing the complete bit is latched.
   // ========================================================================================
   6: NOP();
   // ======================================================================================
   // PART 0: GET NEW RANDOM NUMBER (qa)
   // ======================================================================================
   7: XIC(EdDSA_STATES[3].CMD.0)XIO(EdDSA_STATES[3].DONE.0)[ONS(EdDSA_STATES[3].ONS.0) OTL(PRNG.SEQCTRL_RESET) ,PRNG(PRNG,Temp_Processor_C1,Temp_Processor_D1,Temp_Processor_E1,Temp_Processor_L,Temp_Processor_MSG,Temp_Processor_HASH,PRNG_Constant,PRNG_Seed,PRNG_Counter,PRN) ,XIC(PRNG.SEQCTRL_DN) OTL(EdDSA_STATES[3].DONE.0) ];
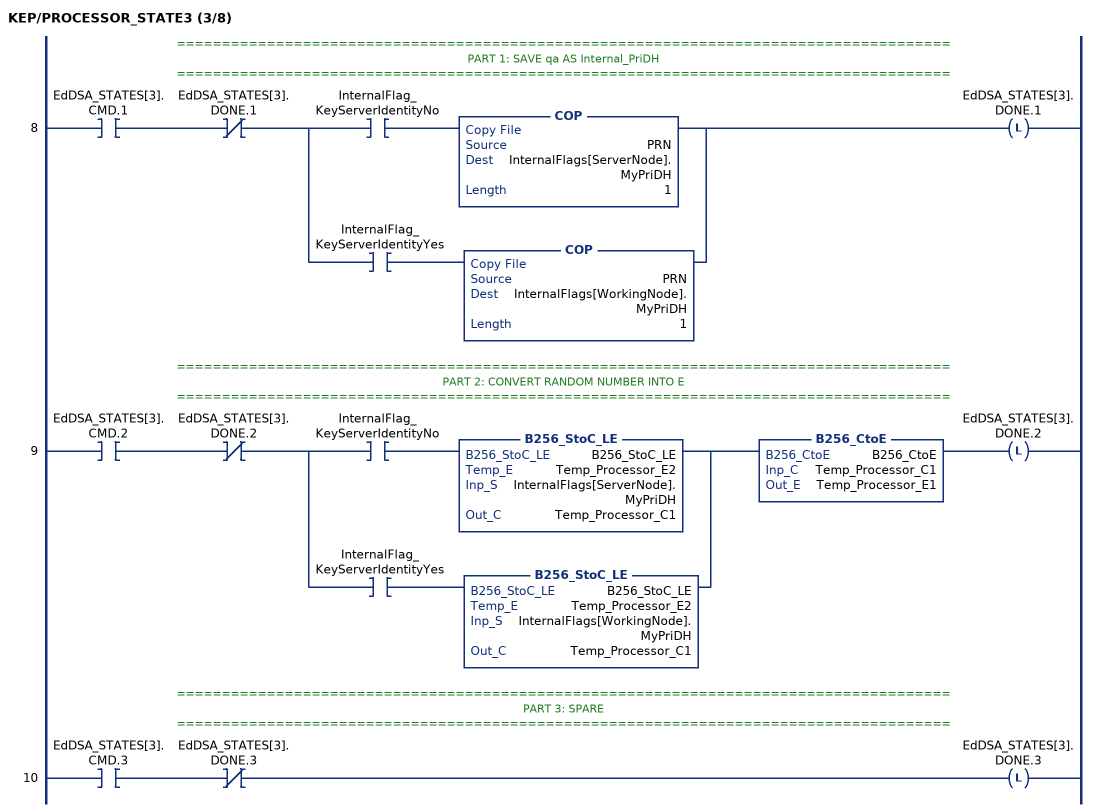
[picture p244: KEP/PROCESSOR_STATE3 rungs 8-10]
   // ======================================================================================
   // PART 1: SAVE qa AS Internal_PriDH
   // ======================================================================================
   8: XIC(EdDSA_STATES[3].CMD.1)XIO(EdDSA_STATES[3].DONE.1)[XIC(InternalFlag_KeyServerIdentityNo) COP(PRN,InternalFlags[ServerNode].MyPriDH,1) ,XIC(InternalFlag_KeyServerIdentityYes) COP(PRN,InternalFlags[WorkingNode].MyPriDH,1) ]OTL(EdDSA_STATES[3].DONE.1);
   // ======================================================================================
   // PART 2: CONVERT RANDOM NUMBER INTO E
   // ======================================================================================
   9: XIC(EdDSA_STATES[3].CMD.2)XIO(EdDSA_STATES[3].DONE.2)[XIC(InternalFlag_KeyServerIdentityNo) B256_StoC_LE(B256_StoC_LE,Temp_Processor_E2,InternalFlags[ServerNode].MyPriDH,Temp_Processor_C1) ,XIC(InternalFlag_KeyServerIdentityYes) B256_StoC_LE(B256_StoC_LE,Temp_Processor_E2,InternalFlags[WorkingNode].MyPriDH,Temp_Processor_C1) ]B256_CtoE(B256_CtoE,Temp_Processor_C1,Temp_Processor_E1)OTL(EdDSA_STATES[3].DONE.2);
   // ======================================================================================
   // PART 3: SPARE
   // ======================================================================================
   10: XIC(EdDSA_STATES[3].CMD.3)XIO(EdDSA_STATES[3].DONE.3)OTL(EdDSA_STATES[3].DONE.3);
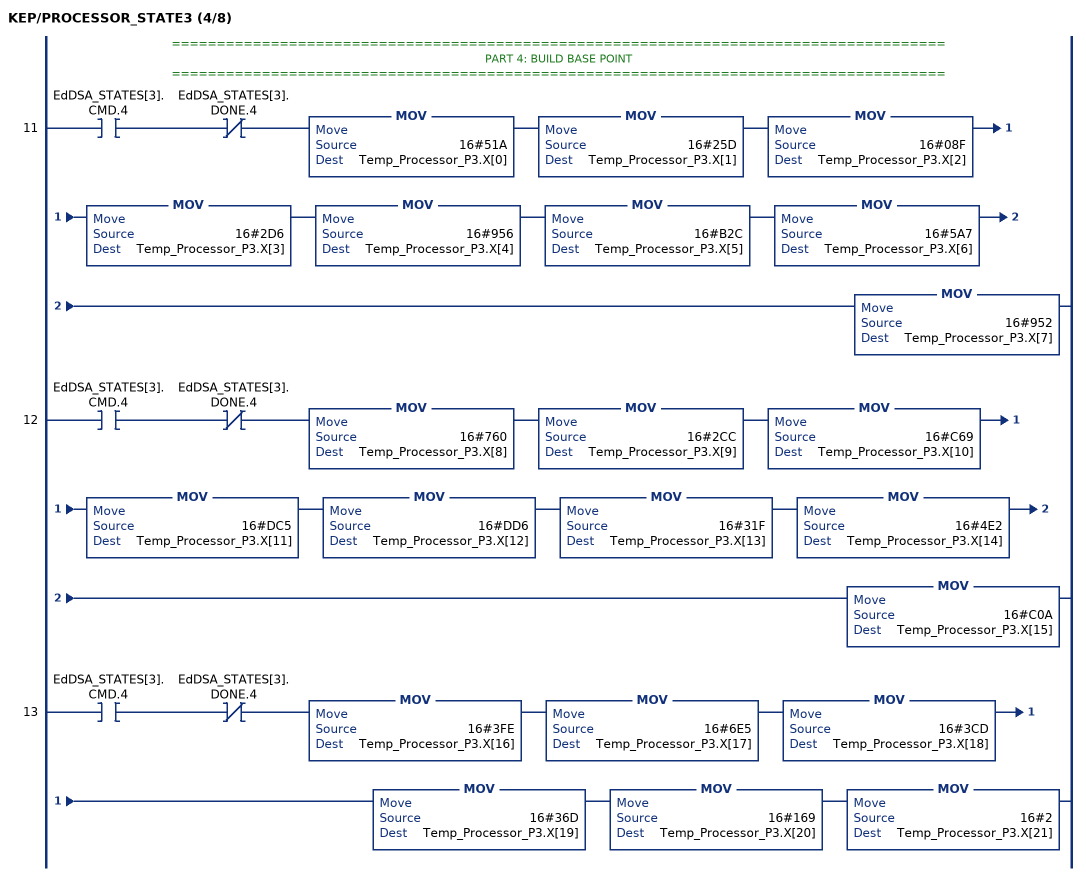
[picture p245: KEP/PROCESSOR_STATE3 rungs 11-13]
   // ======================================================================================
   // PART 4: BUILD BASE POINT
   // ======================================================================================
   11: XIC(EdDSA_STATES[3].CMD.4)XIO(EdDSA_STATES[3].DONE.4)MOV(16#51A,Temp_Processor_P3.X[0])MOV(16#25D,Temp_Processor_P3.X[1])MOV(16#08F,Temp_Processor_P3.X[2])MOV(16#2D6,Temp_Processor_P3.X[3])MOV(16#956,Temp_Processor_P3.X[4])MOV(16#B2C,Temp_Processor_P3.X[5])MOV(16#5A7,Temp_Processor_P3.X[6])MOV(16#952,Temp_Processor_P3.X[7]);
   12: XIC(EdDSA_STATES[3].CMD.4)XIO(EdDSA_STATES[3].DONE.4)MOV(16#760,Temp_Processor_P3.X[8])MOV(16#2CC,Temp_Processor_P3.X[9])MOV(16#C69,Temp_Processor_P3.X[10])MOV(16#DC5,Temp_Processor_P3.X[11])MOV(16#DD6,Temp_Processor_P3.X[12])MOV(16#31F,Temp_Processor_P3.X[13])MOV(16#4E2,Temp_Processor_P3.X[14])MOV(16#C0A,Temp_Processor_P3.X[15]);
   13: XIC(EdDSA_STATES[3].CMD.4)XIO(EdDSA_STATES[3].DONE.4)MOV(16#3FE,Temp_Processor_P3.X[16])MOV(16#6E5,Temp_Processor_P3.X[17])MOV(16#3CD,Temp_Processor_P3.X[18])MOV(16#36D,Temp_Processor_P3.X[19])MOV(16#169,Temp_Processor_P3.X[20])MOV(16#2,Temp_Processor_P3.X[21]);
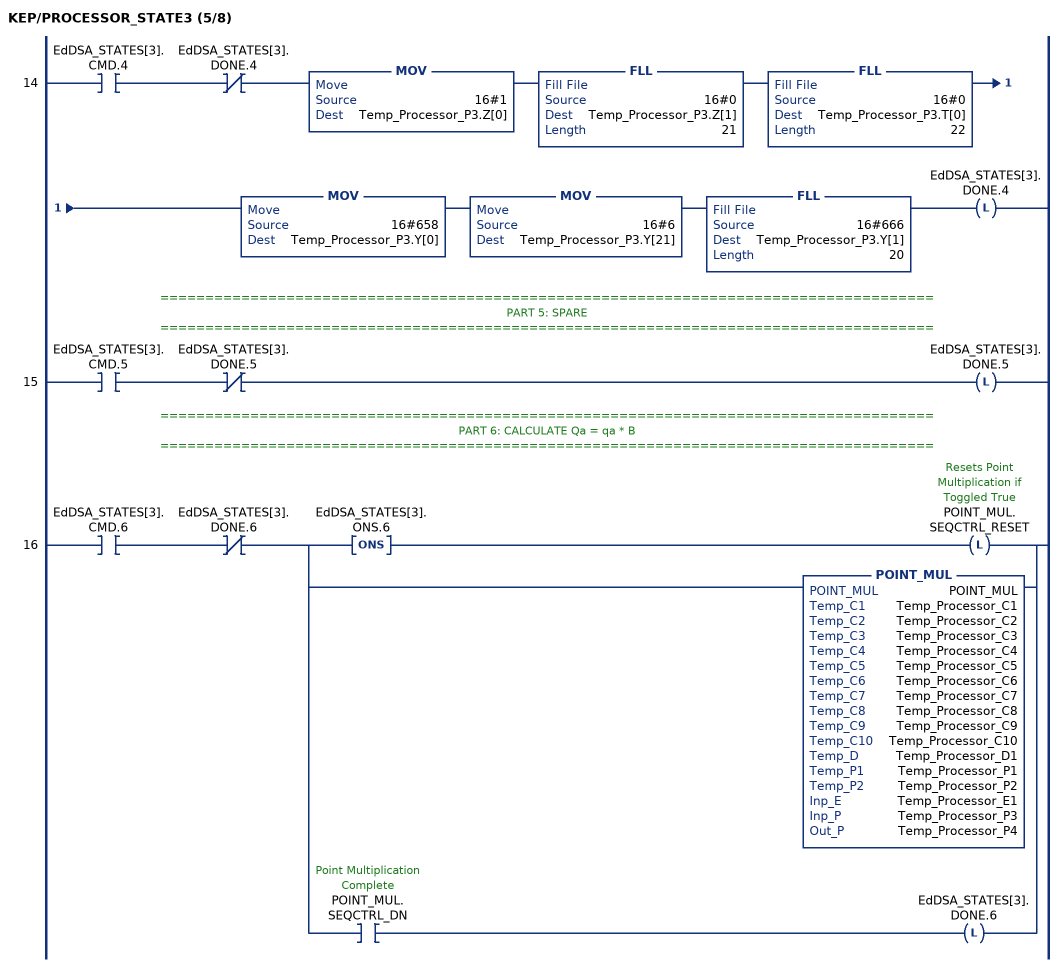
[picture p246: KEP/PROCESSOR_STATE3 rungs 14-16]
   14: XIC(EdDSA_STATES[3].CMD.4)XIO(EdDSA_STATES[3].DONE.4)MOV(16#1,Temp_Processor_P3.Z[0])FLL(16#0,Temp_Processor_P3.Z[1],21)FLL(16#0,Temp_Processor_P3.T[0],22)MOV(16#658,Temp_Processor_P3.Y[0])MOV(16#6,Temp_Processor_P3.Y[21])FLL(16#666,Temp_Processor_P3.Y[1],20)OTL(EdDSA_STATES[3].DONE.4);
   // ======================================================================================
   // PART 5: SPARE
   // ======================================================================================
   15: XIC(EdDSA_STATES[3].CMD.5)XIO(EdDSA_STATES[3].DONE.5)OTL(EdDSA_STATES[3].DONE.5);
   // ======================================================================================
   // PART 6: CALCULATE Qa = qa * B
   // ======================================================================================
   16: XIC(EdDSA_STATES[3].CMD.6)XIO(EdDSA_STATES[3].DONE.6)[ONS(EdDSA_STATES[3].ONS.6) OTL(POINT_MUL.SEQCTRL_RESET) ,POINT_MUL(POINT_MUL,Temp_Processor_C1,Temp_Processor_C2,Temp_Processor_C3,Temp_Processor_C4,Temp_Processor_C5,Temp_Processor_C6,Temp_Processor_C7,Temp_Processor_C8,Temp_Processor_C9,Temp_Processor_C10,Temp_Processor_D1,Temp_Processor_P1,Temp_Processor_P2,Temp_Processor_E1,Temp_Processor_P3,Temp_Processor_P4) ,XIC(POINT_MUL.SEQCTRL_DN) OTL(EdDSA_STATES[3].DONE.6) ];
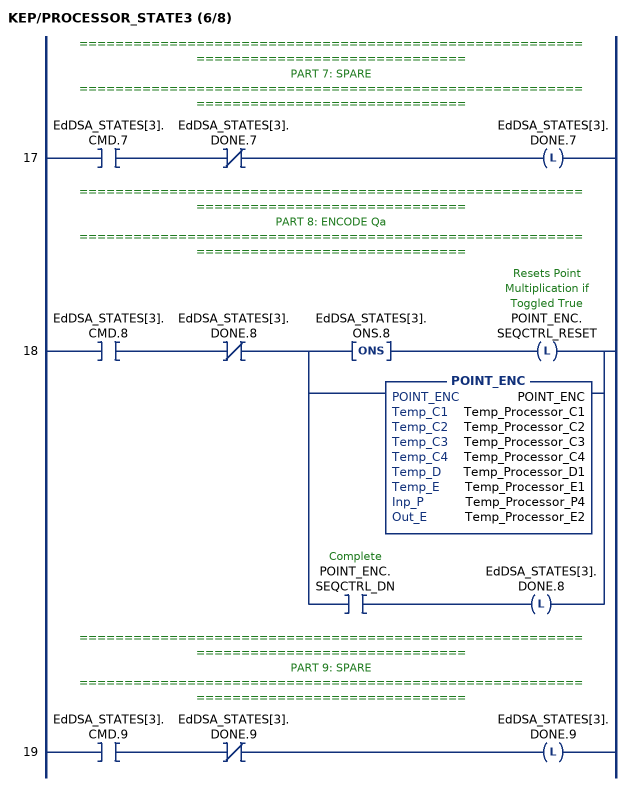
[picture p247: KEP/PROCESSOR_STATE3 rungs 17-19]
   // ======================================================================================
   // PART 7: SPARE
   // ======================================================================================
   17: XIC(EdDSA_STATES[3].CMD.7)XIO(EdDSA_STATES[3].DONE.7)OTL(EdDSA_STATES[3].DONE.7);
   // ======================================================================================
   // PART 8: ENCODE Qa
   // ======================================================================================
   18: XIC(EdDSA_STATES[3].CMD.8)XIO(EdDSA_STATES[3].DONE.8)[ONS(EdDSA_STATES[3].ONS.8) OTL(POINT_ENC.SEQCTRL_RESET) ,POINT_ENC(POINT_ENC,Temp_Processor_C1,Temp_Processor_C2,Temp_Processor_C3,Temp_Processor_C4,Temp_Processor_D1,Temp_Processor_E1,Temp_Processor_P4,Temp_Processor_E2) ,XIC(POINT_ENC.SEQCTRL_DN) OTL(EdDSA_STATES[3].DONE.8) ];
   // ======================================================================================
   // PART 9: SPARE
   // ======================================================================================
   19: XIC(EdDSA_STATES[3].CMD.9)XIO(EdDSA_STATES[3].DONE.9)OTL(EdDSA_STATES[3].DONE.9);
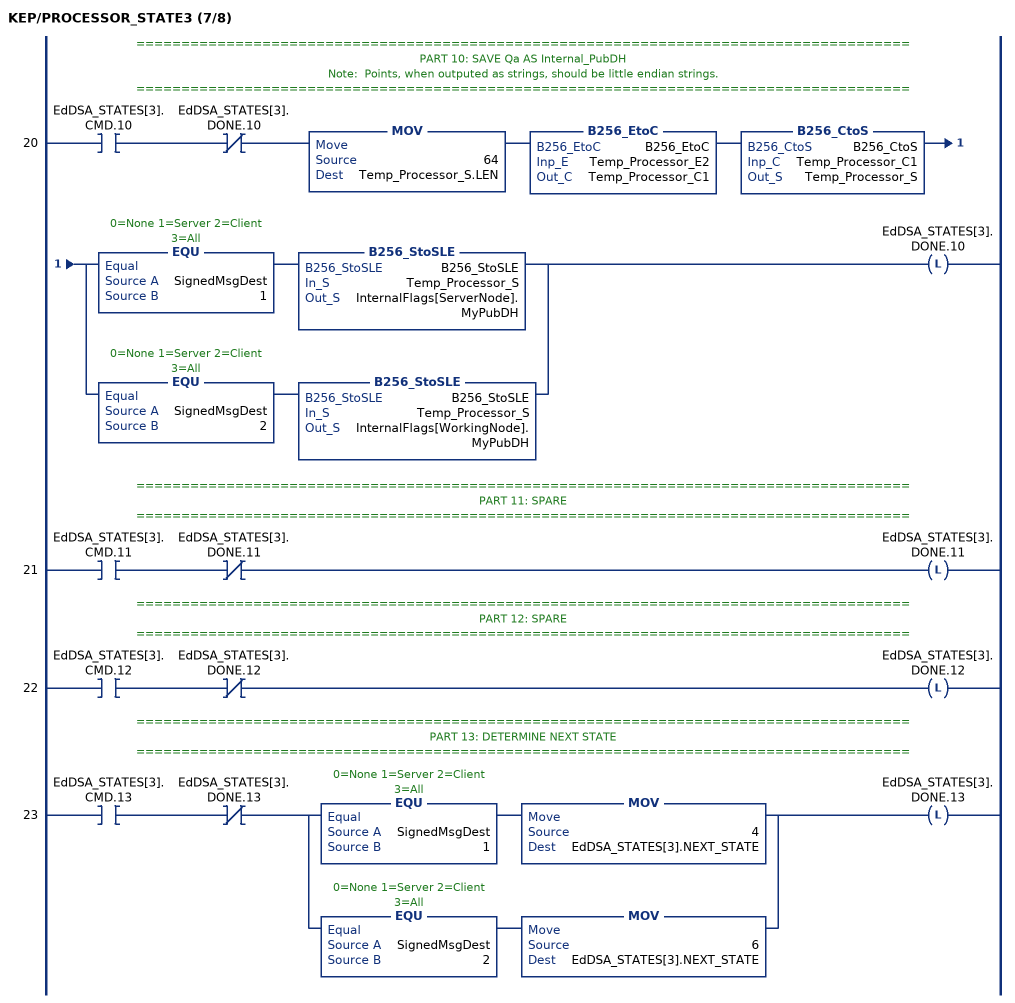
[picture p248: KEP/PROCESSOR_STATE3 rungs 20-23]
   // ======================================================================================
   // PART 10: SAVE Qa AS Internal_PubDH
   // Note:  Points, when outputed as strings, should be little endian strings.
   // ======================================================================================
   20: XIC(EdDSA_STATES[3].CMD.10)XIO(EdDSA_STATES[3].DONE.10)MOV(64,Temp_Processor_S.LEN)B256_EtoC(B256_EtoC,Temp_Processor_E2,Temp_Processor_C1)B256_CtoS(B256_CtoS,Temp_Processor_C1,Temp_Processor_S)[EQU(SignedMsgDest,1) B256_StoSLE(B256_StoSLE,Temp_Processor_S,InternalFlags[ServerNode].MyPubDH) ,EQU(SignedMsgDest,2) B256_StoSLE(B256_StoSLE,Temp_Processor_S,InternalFlags[WorkingNode].MyPubDH) ]OTL(EdDSA_STATES[3].DONE.10);
   // ======================================================================================
   // PART 11: SPARE
   // ======================================================================================
   21: XIC(EdDSA_STATES[3].CMD.11)XIO(EdDSA_STATES[3].DONE.11)OTL(EdDSA_STATES[3].DONE.11);
   // ======================================================================================
   // PART 12: SPARE
   // ======================================================================================
   22: XIC(EdDSA_STATES[3].CMD.12)XIO(EdDSA_STATES[3].DONE.12)OTL(EdDSA_STATES[3].DONE.12);
   // ======================================================================================
   // PART 13: DETERMINE NEXT STATE
   // ======================================================================================
   23: XIC(EdDSA_STATES[3].CMD.13)XIO(EdDSA_STATES[3].DONE.13)[EQU(SignedMsgDest,1) MOV(4,EdDSA_STATES[3].NEXT_STATE) ,EQU(SignedMsgDest,2) MOV(6,EdDSA_STATES[3].NEXT_STATE) ]OTL(EdDSA_STATES[3].DONE.13);
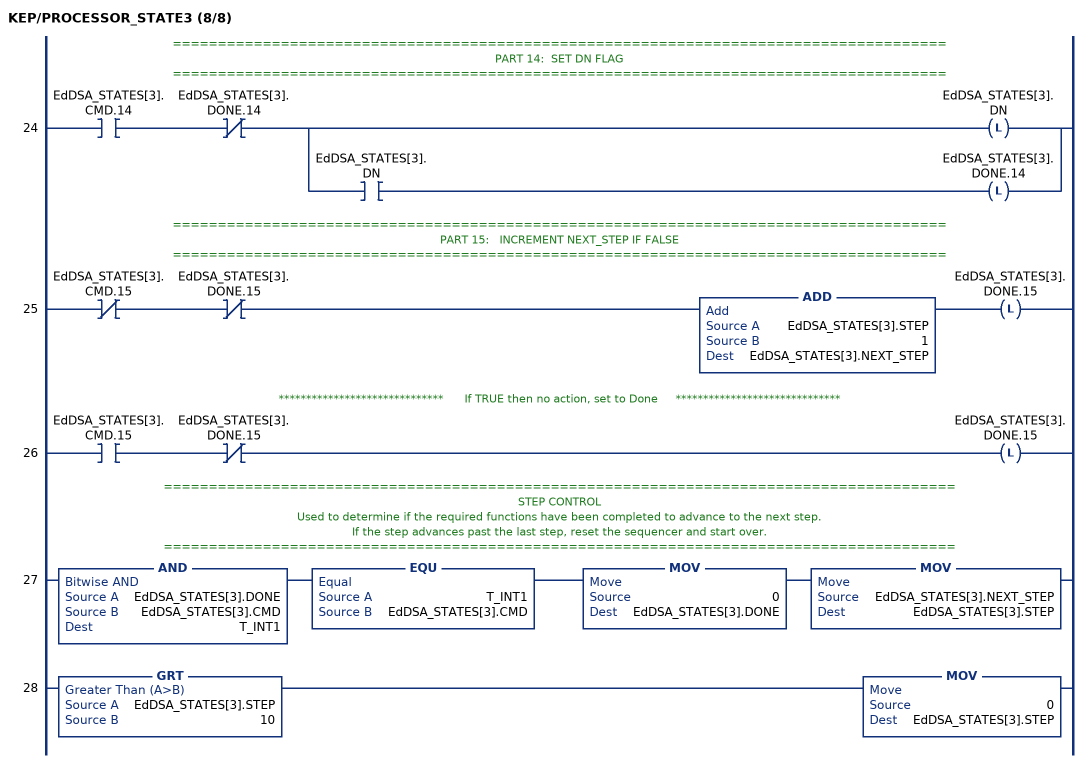
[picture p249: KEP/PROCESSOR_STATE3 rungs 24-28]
   // ======================================================================================
   // PART 14:  SET DN FLAG
   // ======================================================================================
   24: XIC(EdDSA_STATES[3].CMD.14)XIO(EdDSA_STATES[3].DONE.14)[OTL(EdDSA_STATES[3].DN) ,XIC(EdDSA_STATES[3].DN) OTL(EdDSA_STATES[3].DONE.14) ];
   // ======================================================================================
   // PART 15:   INCREMENT NEXT_STEP IF FALSE
   // ======================================================================================
   25: XIO(EdDSA_STATES[3].CMD.15)XIO(EdDSA_STATES[3].DONE.15)ADD(EdDSA_STATES[3].STEP,1,EdDSA_STATES[3].NEXT_STEP)OTL(EdDSA_STATES[3].DONE.15);
   // ******************************      If TRUE then no action, set to Done     ******************************
   26: XIC(EdDSA_STATES[3].CMD.15)XIO(EdDSA_STATES[3].DONE.15)OTL(EdDSA_STATES[3].DONE.15);
   // ========================================================================================
   // STEP CONTROL
   // Used to determine if the required functions have been completed to advance to the next step.
   // If the step advances past the last step, reset the sequencer and start over.
   // ========================================================================================
   27: AND(EdDSA_STATES[3].DONE,EdDSA_STATES[3].CMD,T_INT1)EQU(T_INT1,EdDSA_STATES[3].CMD)MOV(0,EdDSA_STATES[3].DONE)MOV(EdDSA_STATES[3].NEXT_STEP,EdDSA_STATES[3].STEP);
   28: GRT(EdDSA_STATES[3].STEP,10)MOV(0,EdDSA_STATES[3].STEP);
END_ROUTINE
